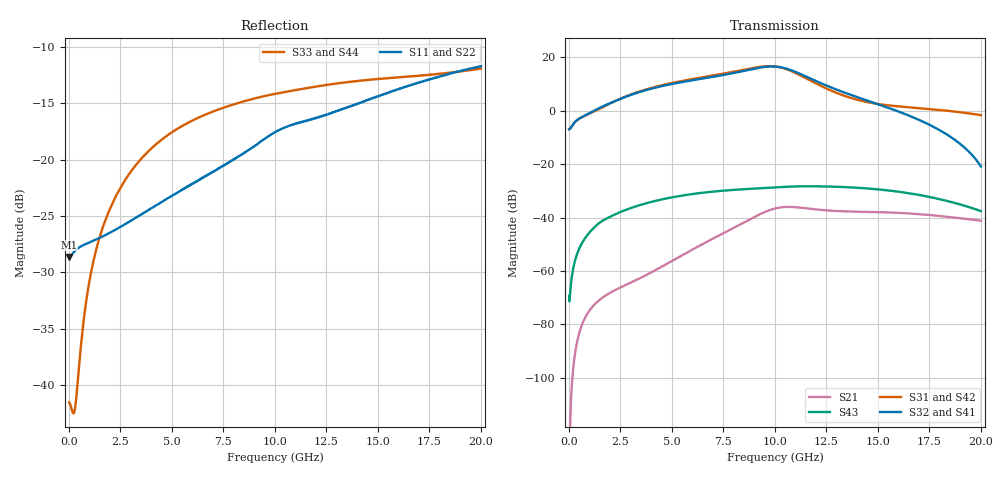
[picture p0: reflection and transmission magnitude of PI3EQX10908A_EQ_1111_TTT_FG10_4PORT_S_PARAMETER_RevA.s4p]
! NPort=4 DATA=2000 NOISE=0 GROUPDELAY=0 COMPLEX_DATAFORMAT=POLAR
! NumOfBlock=1 NumOfParam=0
! .MODEL Smodel S TSTONEFILE=PI3EQX10908A_EQ_1111_TTT_FG10_4PORT_S_PARAMETER_RevA.s4p TYPE=S
!  -- The above .MODEL line can be used for the S element in the netlist.
! The s parameter is extracted from the linear redriver, it is not bi-directional; only s(4,1)s(4,2) and s(3,1)s(3,2)
! should be the insertion loss
!Port definition:
!Port1 = input+
!Port2 = input-
!Port3 = output+
!Port4 = output-
# Hz S MA R  50
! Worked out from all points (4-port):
!   2000 points, 10 MHz to 20 GHz, reference 50 ohm
!   strongest paths, dB at 10 MHz, 5.01 GHz, 10.01 GHz, 15.01 GHz, 20 GHz:
!     S32: -6.9, 10.0, 16.5, 2.4, -20.9
!     S41: -6.9, 10.0, 16.5, 2.4, -20.8
!     S31: -6.9, 10.4, 16.6, 2.5, -1.7
!     S42: -6.9, 10.4, 16.6, 2.5, -1.7
!     S43: -69.4, -32.4, -28.7, -29.5, -37.6
!     S21: -127.2, -56.2, -36.6, -38.0, -41.2
!   lowest |S11| = -28.6 dB at 10 MHz (marker M1), VSWR 1.08, Z = 46.4 - j0.024 ohm
!   |S11| at or under -10 dB: start of sweep to end of sweep
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1e7  0.03701 -179.6  4.341e-07 14.7  0 0.0  0 0.0
     4.341e-07 14.7  0.03701 -179.6  0 0.0  0 0.0
     0.4506 1.2  0.4506 -178.8  0.008374 26.0  0.00034 -27.1
     0.4506 -178.8  0.4506 1.2  0.00034 -27.1  0.008374 26.0
6.27e9  0.08082 -121.6  0.002867 133.8  2.629e-07 70.0  1.499e-07 140.8
        0.002867 133.9  0.08084 -121.6  1.499e-07 140.8  2.629e-07 70.0
        4.084 -47.3  3.862 126.5  0.1535 16.1  0.0284 21.5
        3.862 126.6  4.084 -47.3  0.0284 21.5  0.1535 16.1
8.89e9  0.1131 -112.2  0.009727 108.5  2.058e-06 23.8  1.312e-06 113.6
        0.00973 108.5  0.1132 -112.2  1.312e-06 113.6  2.058e-06 23.8
        6.266 -111.2  5.997 63.0  0.1859 -5.0  0.0346 -5.9
        5.998 63.0  6.266 -111.2  0.0346 -5.9  0.1859 -5.0
1.025e10  0.1363 -112.3  0.0154 71.0  3.871e-06 -10.9  4.057e-06 79.9
          0.0154 71.0  0.1364 -112.3  4.058e-06 79.9  3.872e-06 -10.9
          6.49 -165.8  6.532 7.6  0.1981 -14.3  0.03712 -19.8
          6.532 7.6  6.49 -165.8  0.03712 -19.8  0.1981 -14.3
1.14e10  0.1479 -113.6  0.01505 40.2  4.97e-06 -22.0  7.293e-06 43.7
         0.01504 40.2  0.148 -113.6  7.296e-06 43.7  4.969e-06 -22.1
         4.251 152.5  4.568 -37.2  0.2069 -21.0  0.03838 -33.4
         4.568 -37.2  4.251 152.5  0.03838 -33.4  0.2069 -21.0
1.36e10  0.1715 -112.0  0.01297 13.0  1.372e-05 -36.0  1.627e-05 -6.2
         0.01296 13.0  0.1715 -112.0  1.627e-05 -6.2  1.371e-05 -36.0
         1.776 121.5  2.033 -85.5  0.2216 -32.5  0.03677 -59.9
         2.032 -85.5  1.776 121.6  0.03677 -59.9  0.2216 -32.5
2e10  0.2603 -115.0  0.008737 -40.3  8.763e-05 -148.3  7.124e-05 -139.7
      0.008733 -40.1  0.2605 -115.1  7.125e-05 -139.7  8.761e-05 -148.3
      0.826 52.1  0.09036 168.7  0.2539 -52.3  0.01319 -136.5
      0.09078 169.2  0.8268 52.1  0.01319 -136.5  0.2539 -52.3
